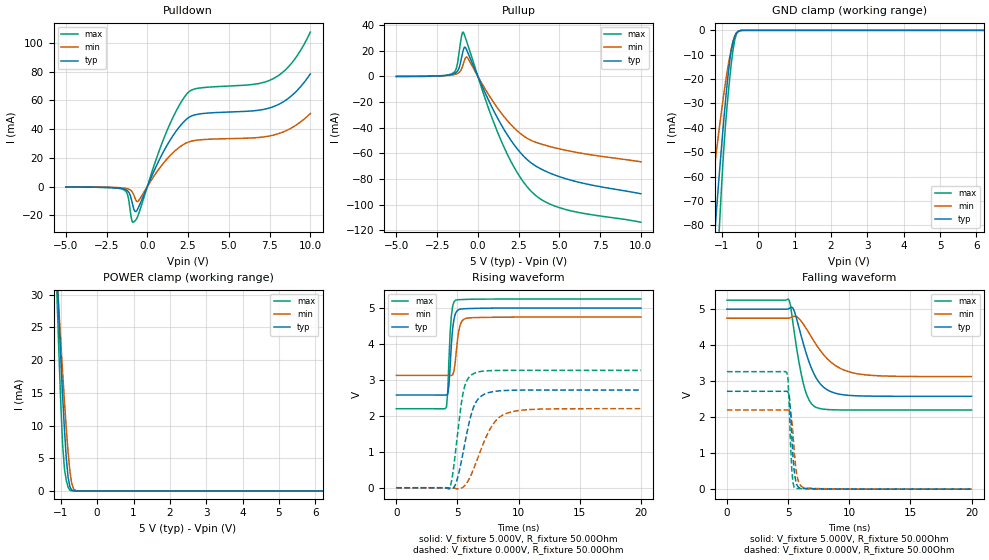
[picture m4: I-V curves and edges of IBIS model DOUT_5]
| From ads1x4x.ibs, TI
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|   DOutput 5.0V Model
[Model]   DOUT_5
Model_type   3-state
|Signals   DOUT_nDRDY
| variable   typ   min   max
|C_comp Output Tri-state
C_comp   3.383pF   4.134pF   2.648pF
|C_comp Output Low
|C_comp   5.617pF   6.618pF   4.944pF
|C_comp Output High
|C_comp   17.151pF   13.353pF   29.975pF
[Model Spec]
|Timing spec test load voltage corners 0.5*VCC
Vmeas   2.5V   2.375V   2.625V
Vref   2.5V   2.375V   2.625V
|Junction Temperature
[Temperature Range]   40.0   105.0   -40.0
[Voltage range]   5.0V   4.75V   5.25V
[pullup reference]   5.0V   4.75V   5.25V
[power clamp reference]   5.0V   4.75V   5.25V
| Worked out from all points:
|   slope of the pulldown table from 0 to 0.75 V, typ, clamps not added: 39.5 ohm
|   slope of the pullup table from 0 to 0.75 V, typ, clamps not added: 35.5 ohm
|   GND clamp passes 1 mA (typ) near -0.60 V on its own axis
|   POWER clamp passes 1 mA (typ) near -0.76 V on its own axis
|   falling waveform, V_fixture 5.000V, R_fixture 50.00Ohm: 20-80 % time 1.47ns typ, 2.25ns min, 960ps max; typ from 5 V to 2.58 V
|   rising waveform, V_fixture 5.000V, R_fixture 50.00Ohm: 20-80 % time 298ps typ, 345ps min, 253ps max; typ from 2.58 V to 5 V
|   rising waveform, V_fixture 0.000V, R_fixture 50.00Ohm: 20-80 % time 1.05ns typ, 1.68ns min, 730ps max; typ from 0 V to 2.72 V
|   falling waveform, V_fixture 0.000V, R_fixture 50.00Ohm: 20-80 % time 292ps typ, 355ps min, 231ps max; typ from 2.72 V to 0 V
[Pulldown]
|   Voltage   I(typ)   I(min)   I(max)
-5V       -197.3uA   -151.9uA   -197.1uA
-1.45V    -1.57mA    -940.8uA   -2.095mA
-1.2V     -2.999mA   -1.479mA   -5.884mA
-950mV    -10.02mA   -3.227mA   -23.39mA
-850mV    -14.64mA   -5.17mA    -24.65mA
-700mV    -17.33mA   -9.318mA   -23.06mA
-550mV    -14.61mA   -10mA      -19.5mA
1.1V      26.57mA    17.87mA    35.97mA
2.45V     47.36mA    30.72mA    64.88mA
7.7V      55.51mA    35.76mA    74.99mA
8.9V      63.77mA    41.23mA    86.6mA
10V       78.43mA    50.89mA    107.5mA
[GND Clamp]
|   Voltage   I(typ)   I(min)   I(max)
-5V       -958.6mA   -692.2mA   -1.337A
-1.4V     -124.9mA   -82.22mA   -180.9mA
-1.35V    -114.4mA   -75.38mA   -165.2mA
-1.2V     -83.67mA   -55.66mA   -118.9mA
-1.15V    -73.79mA   -49.39mA   -103.9mA
-1.1V     -64.11mA   -43.29mA   -89.08mA
-1.05V    -54.69mA   -37.37mA   -74.73mA
-950mV    -36.78mA   -26.21mA   -48.68mA
-800mV    -14.07mA   -11.85mA   -21.67mA
-650mV    -2.397mA   -2.491mA   -3.953mA
-550mV    -339.5uA   -376.7uA   -400.6uA
10V       0A         0A         0A
[Pullup]
|   Voltage   I(typ)   I(min)   I(max)
-5V       -23.11uA   -11.41uA   -36.23uA
-1.5V     1.91mA     1.31mA     2.79mA
-1.3V     3.403mA    2.022mA    7.13mA
-1V       14.67mA    5.853mA    31.59mA
-900mV    20.28mA    9.455mA    34.57mA
-800mV    22.89mA    13.36mA    31.53mA
-650mV    19.51mA    14.81mA    25.83mA
1.35V     -35.84mA   -27.21mA   -47.89mA
2.35V     -55.51mA   -41.76mA   -73.74mA
3.25V     -67.35mA   -49.84mA   -89.42mA
5.35V     -79.71mA   -57.56mA   -103.8mA
10V       -91.58mA   -66.66mA   -113.8mA
[POWER Clamp]
|   Voltage   I(typ)   I(min)   I(max)
-5V       290.3mA    256mA      340.9mA
-1.15V    39.04mA    37.28mA    37.58mA
-1.1V     32.58mA    32.34mA    29.04mA
-1.05V    26.27mA    27.51mA    20.82mA
-1V       20.23mA    22.78mA    13.27mA
-950mV    14.56mA    18.18mA    7.113mA
-900mV    9.406mA    13.76mA    3.405mA
-800mV    2.088mA    5.941mA    579.2uA
-750mV    647.5uA    3.017mA    107.9uA
-650mV    29.24uA    327.1uA    2.074uA
-550mV    1.126uA    18.06uA    52.38nA
10V       0A         0A         0A
[Ramp]
R_load = 50.00Ohm
|   typ   min   max
dV/dt_r   1.631V/1.047ns   1.320V/1.677ns   1.959V/730.007ps
dV/dt_f   1.452V/1.473ns   973.923mV/2.249ns   1.831V/960.316ps
[Falling Waveform]
V_fixture = 5.000V
V_fixture_min = 4.750V
V_fixture_max = 5.250V
R_fixture = 50.00Ohm
|   Time   V(typ)   V(min)   V(max)
0s        5V         4.75V      5.25V
5.1ns     5.025V     4.754V     5.242V
5.5ns     4.954V     4.8V       4.371V
5.9ns     4.478V     4.732V     3.511V
6.3ns     3.98V      4.558V     2.868V
6.8ns     3.457V     4.287V     2.428V
7.3ns     3.088V     4.015V     2.272V
8.4ns     2.725V     3.56V      2.209V
10.5ns    2.595V     3.218V     2.199V
20ns      2.58V      3.127V     2.198V
[Rising Waveform]
V_fixture = 5.000V
V_fixture_min = 4.750V
V_fixture_max = 5.250V
R_fixture = 50.00Ohm
|   Time   V(typ)   V(min)   V(max)
0s        2.58V      3.127V     2.198V
4.1ns     2.579V     3.126V     2.249V
4.2ns     2.619V     3.126V     2.653V
4.3ns     2.84V      3.126V     3.551V
4.5ns     3.991V     3.124V     4.78V
4.7ns     4.668V     3.227V     5.16V
4.9ns     4.891V     3.782V     5.225V
5.2ns     4.966V     4.506V     5.234V
5.8ns     4.984V     4.719V     5.242V
20ns      5V         4.75V      5.25V
[Rising Waveform]
V_fixture = 0.000V
V_fixture_min = 0.000V
V_fixture_max = 0.000V
R_fixture = 50.00Ohm
|   Time   V(typ)   V(min)   V(max)
0s        1.244nV    1.436nV    1.191nV
4.3ns     -13.92mV   98.96uV    -34.72mV
4.6ns     -26.68mV   -1.389mV   363.3mV
4.9ns     151.7mV    -25.8mV    1.177V
5.5ns     1.056V     28.76mV    2.708V
5.8ns     1.576V     152.5mV    3.004V
6.4ns     2.309V     593.3mV    3.189V
7.8ns     2.667V     1.711V     3.26V
9.1ns     2.709V     2.08V      3.265V
20ns      2.718V     2.2V       3.265V
[Falling Waveform]
V_fixture = 0.000V
V_fixture_min = 0.000V
V_fixture_max = 0.000V
R_fixture = 50.00Ohm
|   Time   V(typ)   V(min)   V(max)
0s        2.718V     2.2V       3.265V
4.9ns     2.719V     2.202V     3.24V
5ns       2.701V     2.201V     3.055V
5.1ns     2.596V     2.19V      2.256V
5.3ns     1.509V     1.92V      558.1mV
5.4ns     906.5mV    1.53V      182.8mV
5.6ns     271.3mV    691.9mV    19.02mV
5.9ns     42.58mV    169mV      18.1mV
6.4ns     21.34mV    36.09mV    9.984mV
20ns      1.244nV    1.436nV    1.191nV
